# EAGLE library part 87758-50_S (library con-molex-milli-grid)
HEADER
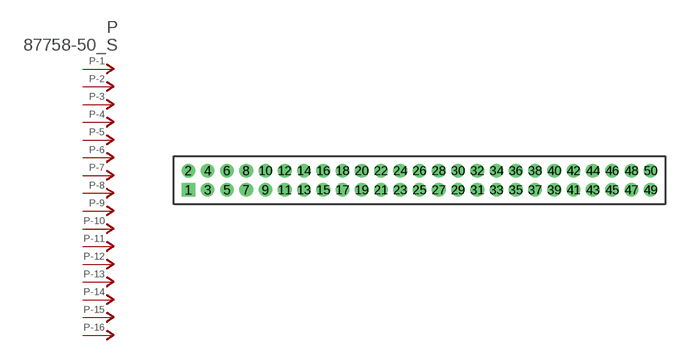
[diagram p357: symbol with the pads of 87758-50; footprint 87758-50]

Designator prefix P; gates -1=P-NV -2=P-N -3=P-N -4=P-N -5=P-N -6=P-N -7=P-N -8=P-N -9=P-N -10=P-N -11=P-N -12=P-N -13=P-N -14=P-N -15=P-N -16=P-N -17=P-N -18=P-N -19=P-N -20=P-N -21=P-N -22=P-N -23=P-N -24=P-N -25=P-N -26=P-N -27=P-N -28=P-N -29=P-N -30=P-N -31=P-N -32=P-N -33=P-N -34=P-N -35=P-N -36=P-N -37=P-N -38=P-N -39=P-N -40=P-N -41=P-N -42=P-N -43=P-N -44=P-N -45=P-N -46=P-N -47=P-N -48=P-N -49=P-N -50=P-N

## 87758-50_S  [87758-50]
1  -1:P  pas
2  -2:P  pas
3  -3:P  pas
4  -4:P  pas
5  -5:P  pas
6  -6:P  pas
7  -7:P  pas
8  -8:P  pas
9  -9:P  pas
10  -10:P  pas
11  -11:P  pas
12  -12:P  pas
13  -13:P  pas
14  -14:P  pas
15  -15:P  pas
16  -16:P  pas
17  -17:P  pas
18  -18:P  pas
19  -19:P  pas
20  -20:P  pas
21  -21:P  pas
22  -22:P  pas
23  -23:P  pas
24  -24:P  pas
25  -25:P  pas
26  -26:P  pas
27  -27:P  pas
28  -28:P  pas
29  -29:P  pas
30  -30:P  pas
31  -31:P  pas
32  -32:P  pas
33  -33:P  pas
34  -34:P  pas
35  -35:P  pas
36  -36:P  pas
37  -37:P  pas
38  -38:P  pas
39  -39:P  pas
40  -40:P  pas
41  -41:P  pas
42  -42:P  pas
43  -43:P  pas
44  -44:P  pas
45  -45:P  pas
46  -46:P  pas
47  -47:P  pas
48  -48:P  pas
49  -49:P  pas
50  -50:P  pas

## Footprint 87758-50 (pad centres in mm)
HEADER Dual Row, Vertical
drill 0.914 square: 1 -24,-1
drill 0.914: 2 -24,1; 3 -22,-1; 4 -22,1; 5 -20,-1; 6 -20,1; 7 -18,-1; 8 -18,1; 9 -16,-1; 10 -16,1; 11 -14,-1; 12 -14,1; 13 -12,-1; 14 -12,1; 15 -10,-1; 16 -10,1; 17 -8,-1; 18 -8,1; 19 -6,-1; 20 -6,1; 21 -4,-1; 22 -4,1; 23 -2,-1; 24 -2,1; 25 0,-1; 26 0,1; 27 2,-1; 28 2,1; 29 4,-1; 30 4,1; 31 6,-1; 32 6,1; 33 8,-1; 34 8,1; 35 10,-1; 36 10,1; 37 12,-1; 38 12,1; 39 14,-1; 40 14,1; 41 16,-1; 42 16,1; 43 18,-1; 44 18,1; 45 20,-1; 46 20,1; 47 22,-1; 48 22,1; 49 24,-1; 50 24,1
